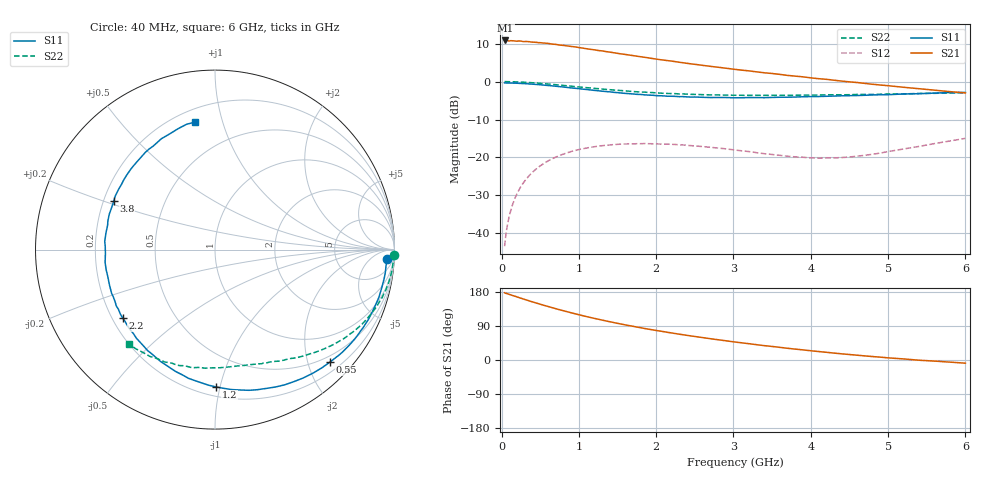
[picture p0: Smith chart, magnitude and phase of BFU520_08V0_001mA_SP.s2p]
! Filename:  P:\Prog\Test\Noise\ATS_data\Testdata_Net\03 Spar\BFU520_APG2013_37_A05_08p0V_001mA_SP_CM01_D.s2p
! Date/Time: Fri 26/Apr/2013 13:00:09
! BFU520_APG2013_37_A05_08p0V_1to20mA_SP_CM01_Bias1_R.s2p
! MDIF S-parameter v. bias file
! BFU520_APG2013_37_A05_08p0V_1to20mA_SP_CM01
! Date/time Tue Apr 23 17:06:44 2013
! bias mode 1
! bias variable = I_out
! VAR bias_var= 1
! VAR V_out= 8.0000
! VAR I_out= 0.9950
! VAR V_in= 0.7890
! VAR I_in= 0.0106
! Device data file deembeded for feedlines and parallel
! Original file: \03 Spar\BFU520_APG2013_37_A05_08p0V_001mA_SP_CM01_R.s2p
! Feed-files: PR047V01_250413_Feed1.s2p, PR047V01_250413_Feed2.s2p
! Parallel-file: PR047V01_250413_Par.s2p
# MHz S MA R 50
!  Freq-MHz  S11-mag  S11-arg  S21-mag  S21-arg  S12-mag  S12-arg  S22-mag  S22-arg
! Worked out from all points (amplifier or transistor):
!   98 points, 40 MHz to 6 GHz, reference 50 ohm
!   highest |S21| = 10.8 dB at 50 MHz (marker M1)
!   |S21| within 3 dB of that: start of sweep to 1.377 GHz
!   unconditionally stable (mu >= 1): 3.52 GHz to 5.192 GHz
!   at 300 MHz: K = 0.08, MSG = 18.4 dB, |S12| = -26.2 dB
!   at 1.6 GHz: K = 0.38, MSG = 11.8 dB, |S12| = -16.4 dB
!   at 6 GHz: K = 0.80, MSG = 6.0 dB, |S12| = -15.0 dB
!   S11 on the Smith chart (normalised r, x): 40 MHz: 17, -23; 550 MHz: 0.38, -2.41; 1.2 GHz: 0.26, -0.97; 2.2 GHz: 0.24, -0.31; 3.8 GHz: 0.24, +0.21; 6 GHz: 0.28, +0.82
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40  0.9598 -3.3  3.464 177.5  0.006794 87.1  0.9973 -1.6
50  0.9585 -4.1  3.476 176.1  0.00845 87.2  0.9989 -2.0
100  0.9574 -8.1  3.423 173.2  0.01682 84.4  0.995 -4.3
120  0.9561 -9.8  3.455 171.8  0.02013 83.4  0.9937 -5.2
200  0.951 -16.3  3.4 166.5  0.0333 79.0  0.9881 -8.7
320  0.9355 -26.1  3.373 158.5  0.05204 72.6  0.9758 -13.9
550  0.8965 -44.2  3.211 144.2  0.08373 61.0  0.9371 -23.0
700  0.8677 -55.5  3.087 135.5  0.1009 54.2  0.909 -28.5
800  0.8478 -62.7  2.991 130.0  0.1109 50.1  0.8883 -31.8
1050  0.7948 -79.8  2.757 117.0  0.1303 40.3  0.84 -39.5
1200  0.7652 -89.6  2.619 109.8  0.1385 35.1  0.813 -43.6
1600  0.698 -113.2  2.276 92.7  0.1505 23.4  0.7524 -53.2
1850  0.6684 -126.5  2.086 83.2  0.1526 17.5  0.7252 -58.2
2050  0.6503 -136.5  1.942 76.4  0.1503 13.5  0.7043 -62.2
2200  0.6403 -143.6  1.858 71.4  0.149 10.9  0.6948 -64.9
2700  0.6159 -165.8  1.586 56.2  0.1361 4.6  0.6676 -74.0
3100  0.6116 178.7  1.415 45.5  0.1226 3.0  0.6592 -80.8
3800  0.6252 154.5  1.178 28.8  0.1019 9.7  0.6603 -93.0
4100  0.6351 145.1  1.091 22.4  0.0981 16.4  0.6634 -98.2
4700  0.6596 128.6  0.9455 10.8  0.1068 31.2  0.6772 -108.8
5200  0.6862 115.8  0.8407 2.9  0.1294 39.0  0.6873 -117.8
6000  0.7189 98.8  0.7085 -8.4  0.1785 41.1  0.7117 -132.4
